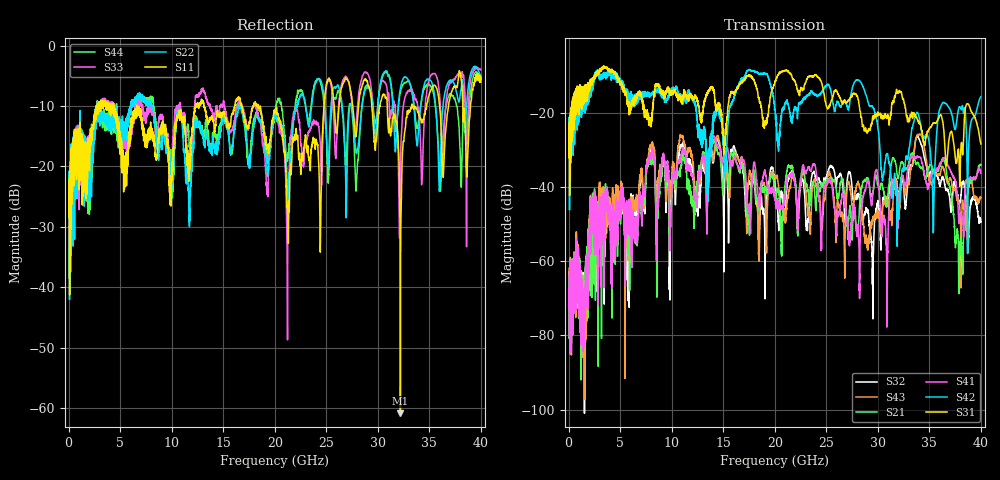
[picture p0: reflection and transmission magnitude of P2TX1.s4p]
!Agilent Technologies,N5245A,MY49151084,A.09.20.08
!Agilent N5245A: A.09.20.08
!Date: Thursday, March 01, 2012 13:58:27
!Correction: S11(Full 4 Port(1,2,3,4))
!S12(Full 4 Port(1,2,3,4))
!S13(Full 4 Port(1,2,3,4))
!S14(Full 4 Port(1,2,3,4))
!S21(Full 4 Port(1,2,3,4))
!S22(Full 4 Port(1,2,3,4))
!S23(Full 4 Port(1,2,3,4))
!S24(Full 4 Port(1,2,3,4))
!S31(Full 4 Port(1,2,3,4))
!S32(Full 4 Port(1,2,3,4))
!S33(Full 4 Port(1,2,3,4))
!S34(Full 4 Port(1,2,3,4))
!S41(Full 4 Port(1,2,3,4))
!S42(Full 4 Port(1,2,3,4))
!S43(Full 4 Port(1,2,3,4))
!S44(Full 4 Port(1,2,3,4))
!S4P File: Measurements: <S11,S12,S13,S14>,
!<S21,S22,S23,S24>,
!<S31,S32,S33,S34>,
!<S41,S42,S43,S44>:
# Hz S  dB  R 50
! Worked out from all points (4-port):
!   3996 points, 50 MHz to 40 GHz, reference 50 ohm
!   strongest paths, dB at 50 MHz, 10.04 GHz, 20.03 GHz, 30.02 GHz, 40 GHz:
!     S31: -27.2, -14.2, -11.5, -20.3, -28.4
!     S42: -25.3, -13.6, -19.2, -24.3, -15.7
!     S41: -63.5, -40.2, -42.9, -37.9, -36.4
!     S21: -64.2, -41.4, -42.0, -39.0, -34.1
!     S43: -61.9, -36.2, -37.9, -47.0, -42.8
!     S32: -62.7, -39.8, -39.6, -44.3, -49.4
!   lowest |S11| = -60.8 dB at 32.19 GHz (marker M1), VSWR 1.00, Z = 49.9 + j0.0361 ohm
!   |S11| at or under -10 dB: 6.651 GHz to 12.3 GHz (5.647 GHz wide, 59.6 % of centre); 13.15 GHz to 16.12 GHz (2.967 GHz wide, 20.3 % of centre); 18.4 GHz to 24.78 GHz (6.378 GHz wide, 29.5 % of centre)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
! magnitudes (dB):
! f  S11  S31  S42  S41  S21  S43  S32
! 50 MHz  -25.3  -27.2  -25.3  -63.5  -64.2  -61.9  -62.7
! 8.02 GHz  -14.2  -21.5  -15.1  -31.5  -33.8  -28.9  -30.7
! 13.56 GHz  -12.7  -14.3  -38.8  -36.0  -37.3  -33.1  -32.7
! 28.09 GHz  -11.0  -16.5  -11.2  -50.9  -51.1  -38.5  -42.3
! 32.19 GHz  -60.8  -14.4  -40.2  -39.4  -34.1  -42.7  -40.8
! 38.01 GHz  -4.5  -33.2  -18.6  -47.4  -55.7  -48.3  -43.9
! 40 GHz  -6.0  -28.4  -15.7  -36.4  -34.1  -42.8  -49.4
